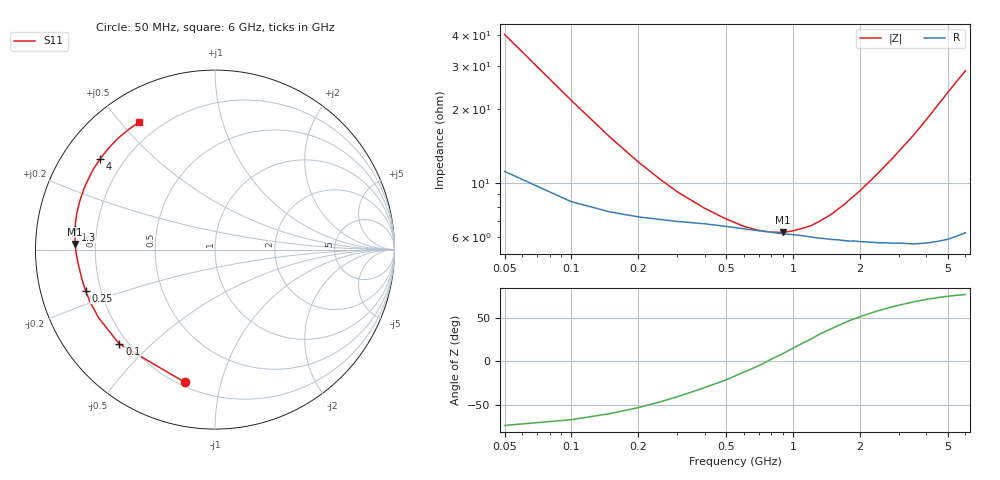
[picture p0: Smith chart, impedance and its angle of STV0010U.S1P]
! SIEMENS Discrete & RF Semiconductors
! BA892
! Si PIN Diode in SCD-80
! IF = 0.01 mA
! S-Parameters:  September  1997
# GHz  S  MA  R  50
!  f  S11
! GHz  MAG  ANG
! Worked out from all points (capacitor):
!   34 points, 50 MHz to 6 GHz, reference 50 ohm
!   read as one part to ground: C = 78.2 pF near 50 MHz
!   lowest |Z| = 6.27 ohm at 900 MHz (marker M1)
!   series resonance near 765 MHz, so ESL is about 550 pH
!   S11 on the Smith chart (normalised r, x): 50 MHz: 0.22, -0.78; 100 MHz: 0.17, -0.40; 250 MHz: 0.14, -0.15; 1.3 GHz: 0.12, +0.07; 4 GHz: 0.11, +0.34; 6 GHz: 0.13, +0.56
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0.05  0.7584 -102.7
0.1  0.7485 -135.4
0.15  0.7516 -149.6
0.2  0.7547 -157.4
0.25  0.7566 -162.4
0.3  0.7588 -166.0
0.4  0.7618 -170.8
0.5  0.7663 -174.0
0.6  0.7703 -176.7
0.7  0.774 -178.7
0.8  0.7768 179.3
0.9  0.7797 177.7
1.1  0.7834 174.6
1.2  0.786 173.3
1.3  0.7883 171.8
1.5  0.7915 169.3
1.6  0.7925 168.0
1.8  0.7956 165.5
2  0.7975 163.3
2.4  0.8017 158.8
2.8  0.8053 154.5
3  0.8066 152.3
3.5  0.8122 147.1
4  0.8159 141.6
4.5  0.8192 136.1
5  0.8225 130.8
5.5  0.8243 125.7
6  0.8265 121.0
